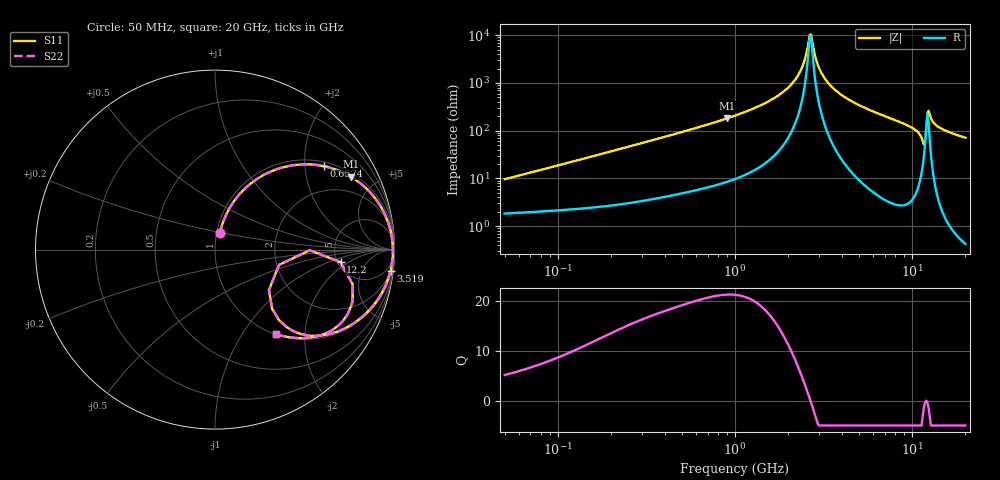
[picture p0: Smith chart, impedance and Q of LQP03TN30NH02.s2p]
!Murata Part Number: LQP03TN30NH02
!These Parameters are Measured in Series Mode Connection
!  o--[Z]--o
!Port1  Port2
!  o-------o
!Freq. Start=50[MHz] Stop=20[GHz], 401[Steps]
# Hz S RI R 50
!Freq.(Hz) S11(Real) S11(Imag) S21(Real) S21(Imag) S12(Real) S12(Imag) S22(Real) S22(Imag)
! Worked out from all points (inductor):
!   401 points, 50 MHz to 20 GHz, reference 50 ohm
!   read as one part in series: L = 29.9 nH near 51.52 MHz
!   highest Q = 21.3 at 900.5 MHz (marker M1), where L = 32 nH
!   self-resonance near 2.647 GHz
!   S11 on the Smith chart (normalised r, x): 50 MHz: 1.04, +0.19; 657.4 MHz: 1.12, +2.51; 3.519 GHz: 2, -17; 12.2 GHz: 5.31, -1.46; 20 GHz: 1.01, -1.43
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5e7  0.0265 0.0905  0.9735 -0.0905  0.9735 -0.0905  0.0265 0.0905
1.364002e8  0.0791 0.2275  0.9209 -0.2275  0.9209 -0.2275  0.0791 0.2275
3.721004e8  0.3314 0.4432  0.6686 -0.4432  0.6686 -0.4432  0.3314 0.4432
6.574395e8  0.607 0.4646  0.393 -0.4646  0.393 -0.4646  0.607 0.4646
9.00459e8  0.7566 0.4064  0.2434 -0.4064  0.2434 -0.4064  0.7566 0.4064
1e9  0.8001 0.3772  0.1999 -0.3772  0.1999 -0.3772  0.8001 0.3772
1.498439e9  0.9263 0.2351  0.0737 -0.2351  0.0737 -0.2351  0.9263 0.2351
1.99176e9  0.9741 0.1209  0.0259 -0.1209  0.0259 -0.1209  0.9741 0.1209
2.348516e9  0.9874 0.0528  0.0126 -0.0528  0.0126 -0.0528  0.9874 0.0528
2.647493e9  0.9909 0.00292  0.00912 -0.00292  0.00912 -0.00292  0.9909 0.00292
2.728004e9  0.9909 -0.0096  0.00906 0.0096  0.00906 0.0096  0.9909 -0.0096
2.98453e9  0.9891 -0.0472  0.0109 0.0472  0.0109 0.0472  0.9891 -0.0472
3.519108e9  0.978 -0.1164  0.022 0.1164  0.022 0.1164  0.978 -0.1164
4.748272e9  0.9294 -0.2417  0.0706 0.2417  0.0706 0.2417  0.9294 -0.2417
7.442007e9  0.7706 -0.4119  0.2294 0.4119  0.2294 0.4119  0.7706 -0.4119
1.050288e10  0.5099 -0.4769  0.4901 0.4769  0.4901 0.4769  0.5099 -0.4769
1.149051e10  0.3183 -0.3298  0.6817 0.3298  0.6817 0.3298  0.3183 -0.3298
1.183995e10  0.3572 -0.0851  0.6428 0.0851  0.6428 0.0851  0.3572 -0.0851
1.220001e10  0.6993 -0.0694  0.3007 0.0694  0.3007 0.0694  0.6993 -0.0694
1.257102e10  0.7659 -0.2916  0.2341 0.2916  0.2341 0.2916  0.7659 -0.2916
1.375312e10  0.6166 -0.4672  0.3834 0.4672  0.3834 0.4672  0.6166 -0.4672
2e10  0.3391 -0.4704  0.6609 0.4704  0.6609 0.4704  0.3391 -0.4704
